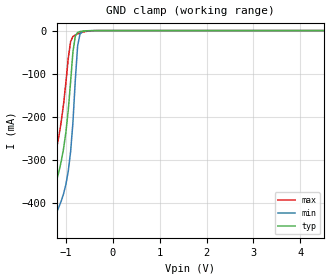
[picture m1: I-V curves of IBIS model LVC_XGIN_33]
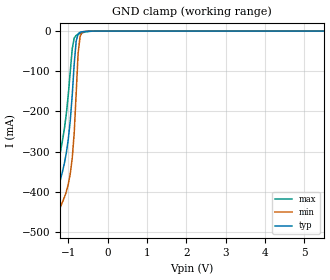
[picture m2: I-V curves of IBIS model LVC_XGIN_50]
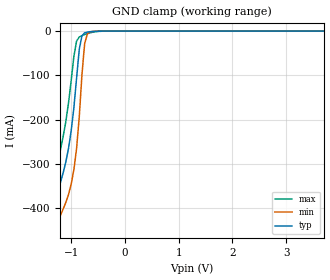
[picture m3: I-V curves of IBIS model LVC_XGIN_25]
| Philips Semiconductors Inc.
| Logic Products Group
| IBIS model of 74LVC2G04
| 3.3V DUAL INVERTER
|[Packages]:
|[Package1]: SOT363 (SC88) 6-pin Package ;
|[Package2]: SOT457 (SC74) 6-pin Package ;
[IBIS Ver]   3.2
[File Name]   lvc2g04.ibs
[File Rev]   1.0
[Date]   31-Jul-2003
[Source]   File created from simulations by LPG
   Philips Semiconductors Nijmegen
[Notes]   V1.0   Ibis model.
| Revision History
| Version Date   Author/ Description
|   Editor
| 1.0   July   2003 RM   Initial Version
| Remarks:
| 1. The Power Clamp curves have been omitted since there is no power clamp
|   diode.
| 2. Non-monotonic sections below 0V in pulldown and pullup curves have been
|   removed (if any).
[Disclaimer]
   (C) Copyright 2003 Philips Semiconductors
   All rights reserved
   Philips Semiconductors warrants and represents that the IBIS model
   identified herein is owned by Philips Semiconductors (PHILIPS). The
   model provided is not warranted as fully representing all of the
   operating characteristics and specifications of the semiconductor
   products to which the model relates.  Moreover, unless there is a
   signed, written agreement to the contrary, this IBIS model is
   furnished on an "as is" basis without support or warranty of any
   kind, either expressed or implied, regarding the use thereof, and
   PHILIPS specifically disclaims all implied warranties of
   merchantability and fitness of the model for any purpose.
   PHILIPS does not assume any liability arising out of the application
   or use of this IBIS model including infringement of patents and
   copyrights, nor does PHILIPS convey any license under its patents and
   copyrights or the rights of others.
   PHILIPS provides IBIS models as a service to our customers. You and
   your company shall not distribute, convey, sell, or give these models
   to anyone else without receiving prior written permission from
   PHILIPS.
   PHILIPS reserves the right to make changes without notice to these
   IBIS models to improve reliability, function, or design.
   Please be aware that your receipt and subsequent use of the IBIS
   information provided shall serve as acceptance of the terms and
   conditions of this agreement.  If you do not accept these terms,
   you should return or destroy the IBIS models and any other
   accompanying information immediately.
|   Info for  SOT363 (SC88) 6-pin Package
[Component]   74LVC2G04_1
[Manufacturer]   Philips Semiconductors Inc.
[package]
|   typ   min   max
R_pkg   4.3700E-02  3.4546E-02   5.2375E-02
L_pkg   1.039E-09   7.420E-10   1.463E-09
C_pkg   1.09E-13   9.20E-14   1.16E-13
[Pin] signal_name   model_name   R_pin   L_pin   C_pin
   1   A1   lvc_xgin 4.48E-02  7.42E-10  1.11E-13
   2   GND   GND 3.74E-02 1.237E-09  1.06E-13
   3   A2   lvc_xgin 4.26E-02  9.37E-10  1.11E-13
   4   Y2#   lvc_xgouti 5.05E-02  9.89E-10  1.16E-13
   5   VCC   POWER 3.45E-02  8.63E-10  9.20E-14
   6   Y1#   lvc_xgouti 5.24E-02 1.463E-09  1.15E-13
|   Info for  SOT457 (SC74) 6-pin Package
[Component]   74LVC2G04_2
[Manufacturer]   Philips Semiconductors Inc.
[package]
|   typ   min   max
R_pkg   6.7794E-02  5.2100E-02   9.3074E-02
L_pkg   1.185E-09   9.680E-10   1.443E-09
C_pkg   1.24E-13   1.09E-13   1.36E-13
[Pin] signal_name   model_name   R_pin   L_pin   C_pin
   1   A1   lvc_xgin 5.21E-02  1.06E-09  1.23E-13
   2   GND   GND 5.86E-02  1.19E-09  1.36E-13
   3   A2   lvc_xgin 8.27E-02 1.325E-09  1.35E-13
   4   Y2#   lvc_xgouti 9.31E-02 1.443E-09  1.27E-13
   5   VCC   POWER 5.26E-02  9.68E-10  1.09E-13
   6   Y1#   lvc_xgouti 6.77E-02 1.123E-09  1.16E-13
[Model Selector]   lvc_xgin
| Remark: If your software does not support the Model Selector
|   Please comment out the lines of the Model Selector, which
|   contain the name of the Model, except the one you want to use.
LVC_XGIN_33   3.3V-Vcc input model
LVC_XGIN_50   5.0V-Vcc input model
LVC_XGIN_25   2.5V-Vcc input model
LVC_XGIN_18   1.8V-Vcc input model
[Model Selector]   lvc_xgouti
| Remark: If your software does not support the Model Selector
|   Please comment out the lines of the Model Selector, which
|   contain the name of the Model, except the one you want to use.
LVC_XGOUTI_33   3.3V-Vcc output model (inverting)
LVC_XGOUTI_50   5.0V-Vcc output model (inverting)
LVC_XGOUTI_25   2.5V-Vcc output model (inverting)
LVC_XGOUTI_18   1.8V-Vcc output model (inverting)
| Models and submodels in the file (8): LVC_XGIN_33 (Input), LVC_XGIN_50 (Input), LVC_XGIN_25 (Input), LVC_XGIN_18 (Input), LVC_XGOUTI_33 (Output), LVC_XGOUTI_50 (Output), LVC_XGOUTI_25 (Output), LVC_XGOUTI_18 (Output)
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|   Model LVC_XGIN_33
[Model]   LVC_XGIN_33
Model_type   Input
Vinl =   0.8V
Vinh =   2.0V
C_comp   2.96pF   2.12pF   3.91pF
[Model Spec]
| Note: The input and output voltage ratings may be exceeded if the input and
|   output current ratings are observed (please refer to the data sheet)
|   Subparameter   typ   min   max
| Thresholds
Vinh   2.0   2.0   2.0
Vinl   0.8   0.8   0.8
| Overshoot
S_overshoot_high   6.5   6.5   6.5   | Static overshoot
S_overshoot_low   -0.5   -0.5   -0.5
D_overshoot_high   7.2   7.2   7.2   | Dynamic overshoot
D_overshoot_low   -0.95   -0.9   -1.0
D_overshoot_time   3n   3n   3n
|Ambient temperature:   25   85   -40
[Temperature Range]   50   105   -10
[Voltage Range]   3.3V   3.0V   3.6V
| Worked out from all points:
|   GND clamp passes 1 mA (typ) near -0.61 V on its own axis
|Process Range   nominal   slow   fast
[GND_clamp]
| voltage   I(typ)   I(min)   I(max)
-5.5V     -4.562A    -4.619A    -4.506A
-1.45V    -549.4mA   -615.4mA   -482.8mA
-1.4V     -502.2mA   -568.5mA   -435.4mA
-1.35V    -455.9mA   -522.5mA   -388.7mA
-1.3V     -411.6mA   -478.9mA   -343.8mA
-1.1V     -304.2mA   -396.4mA   -212.1mA
-950mV    -185.2mA   -327mA     -64.69mA
-850mV    -49.8mA    -213.4mA   -13.79mA
-750mV    -4.324mA   -35.6mA    -7.884mA
-700mV    -2.27mA    -8.526mA   -5.841mA
-550mV    -593.6uA   -425.2uA   -1.597mA
5.5V      375.8pA    2.471nA    52.76pA
|   Model LVC_XGIN_50
[Model]   LVC_XGIN_50
Model_type   Input
Vinl =   1.5V
Vinh =   3.5V
C_comp   2.89pF   1.97pF   3.94pF
[Model Spec]
| Note: The input and output voltage ratings may be exceeded if the input and
|   output current ratings are observed (please refer to the data sheet)
|   Subparameter   typ   min   max
| Thresholds
Vinh   3.5   3.15   3.85
Vinl   1.5   1.35   1.65
| Overshoot
S_overshoot_high   6.5   6.5   6.5   | Static overshoot
S_overshoot_low   -0.5   -0.5   -0.5
D_overshoot_high   11.0   11.0   11.0   | Dynamic overshoot
D_overshoot_low   -0.95   -0.9   -1.0
D_overshoot_time   3n   3n   3n
|Ambient temperature:   25   85   -40
[Temperature Range]   50   105   -10
[Voltage Range]   5.0V   4.5V   5.5V
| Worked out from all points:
|   GND clamp passes 1 mA (typ) near -0.59 V on its own axis
|Process Range   nominal   slow   fast
[GND_clamp]
| voltage   I(typ)   I(min)   I(max)
-5.5V     -4.585A    -4.637A    -4.534A
-1.45V    -567.8mA   -628.4mA   -505.9mA
-1.4V     -520.6mA   -581.5mA   -458.5mA
-1.3V     -430.1mA   -491.9mA   -367mA
-1.2V     -369.6mA   -437.9mA   -299.9mA
-1.05V    -303mA     -399.7mA   -205.6mA
-950mV    -222.3mA   -354.8mA   -100.4mA
-850mV    -82.04mA   -253.9mA   -17.37mA
-800mV    -24.94mA   -156mA     -10.72mA
-750mV    -6.792mA   -54.58mA   -8.095mA
-700mV    -2.837mA   -13.44mA   -6.14mA
5.5V      1.794nA    5.479nA    963.8pA
|   Model LVC_XGIN_25
[Model]   LVC_XGIN_25
Model_type   Input
Vinl =   0.7V
Vinh =   1.7V
C_comp   3.01pF   2.23pF   3.90pF
[Model Spec]
| Note: The input and output voltage ratings may be exceeded if the input and
|   output current ratings are observed (please refer to the data sheet)
|   Subparameter   typ   min   max
| Thresholds
Vinh   1.7   1.7   1.7
Vinl   0.7   0.7   0.7
| Overshoot
S_overshoot_high   6.5   6.5   6.5   | Static overshoot
S_overshoot_low   -0.5   -0.5   -0.5
D_overshoot_high   7.2   7.2   7.2   | Dynamic overshoot
D_overshoot_low   -0.95   -0.9   -1.0
D_overshoot_time   3n   3n   3n
|Ambient temperature:   25   85   -40
[Temperature Range]   30   90   -35
[Voltage Range]   2.5V   2.3V   2.7V
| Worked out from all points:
|   GND clamp passes 1 mA (typ) near -0.61 V on its own axis
|Process Range   nominal   slow   fast
[GND_clamp]
| voltage   I(typ)   I(min)   I(max)
-5.5V     -4.553A    -4.61A     -4.497A
-1.45V    -543.2mA   -609mA     -477mA
-1.4V     -496.1mA   -562.1mA   -429.6mA
-1.35V    -449.7mA   -516.1mA   -382.9mA
-1.25V    -367.8mA   -436.8mA   -298.4mA
-1.1V     -295.9mA   -387.6mA   -204.4mA
-950mV    -173.1mA   -313.3mA   -57.16mA
-850mV    -41.37mA   -194.3mA   -13.46mA
-750mV    -3.847mA   -28.54mA   -7.836mA
-700mV    -2.146mA   -6.789mA   -5.759mA
-550mV    -554.2uA   -385.7uA   -1.497mA
5.5V      211.8pA    1.646nA    21.33pA
